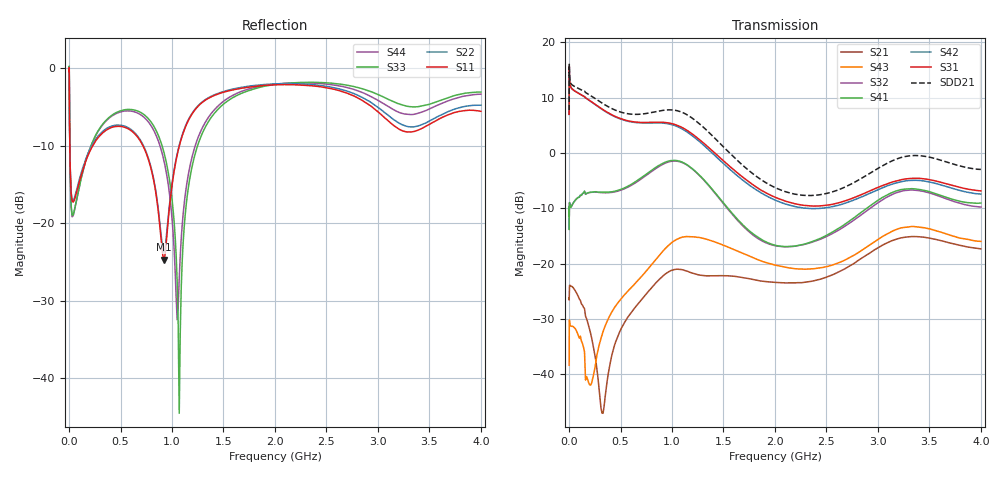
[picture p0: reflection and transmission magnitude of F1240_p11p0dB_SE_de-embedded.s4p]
! Integrated Device Technology
! Corporate Headquarters
! 6024 Silver Creek Valley Road
! San Jose, CA 95138  USA
! Phone:  1-408-284-8200
! Toll Free:  1-800-223-1366
! Webpage:  http://www.idt.com/
! Timing and RF Division
! 515 Groton Road, Suite 102
! Westford, MA 01886-6024
! Device:  F1240
! Description: Dual Intermediate Frequency Digital Variable Gain Amplifier
! Frequency:  10.0 -  500.00 MHz
! Package:  5x5 mm QFN Plastic Package: 32 pin
! Ports:  8 RF, 20 DC
!  Pin  1  = GA3 / Data  Pin 17  = RF OUT_B+
!  Pin  2  = GA4 / CLK  Pin 18  = RF OUT_B-
!  Pin  3  = GA5  Pin 19  = STBY_B
!  Pin  4  = VMODE  Pin 20  = Ground
!  Pin  5  = No Connect  Pin 21  = Ground
!  Pin  6  = GB5  Pin 22  = STB_A
!  Pin  7  = GB4  Pin 23  = RF OUT_A-  = Port 4
!  Pin  8  = GB3  Pin 24  = RF OUT_A+  = Port 3
!  Pin  9  = GB2  Pin 25  = GA0
!  Pin 10  = GB1  Pin 26  = ISET_A
!  Pin 11  = RF IN_B+  Pin 27  = VCC
!  Pin 12  = RF IN_B-  Pin 28  = Ground
!  Pin 13  = Ground  Pin 29  = RF IN_A-  = Port 2
!  Pin 14  = VCC  Pin 30  = RF IN_A+  = Port 1
!  Pin 15  = ISET_B  Pin 31  = GA1
!  Pin 16  = GB0  Pin 32  = GA2 / CSb
! Gain  = +19.5 dB
! State  = 1
! Voltage  = +5.00 V
! Current  = 85.292 mA (one channel only)
! Temperture  =  +25 C
! Test Date  =  2017-10-18
! Board  =  EB4031
! Data:  The device was measured on a custom evaluation board which has
!  individual transmission lines to the RF pins.  Data was collected
!  using a calibrated network analyzer.  The evaluation board was
!  de-embedded using Automatic Fixture Removal.
!  The reference plane is the edge of the package pin.
!  Only Channel A was measured.
!  This data is in single-ended operation.  If your needs are balanced
!  or differential S-parameters then this file needs to be used a
!  linear simulator.
! File Date:  2017-11-10  MJV
! Note:
!  Integrated Device Technology supplies this data as a sample of measured
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# Hz S dB R 100
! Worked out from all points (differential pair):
!   410 points, 500 kHz to 4 GHz, reference 100 ohm
!   strongest paths, dB at 500 kHz, 930 MHz, 1.96 GHz, 2.98 GHz, 4 GHz:
!     S31: 7.0, 5.5, -7.7, -6.4, -6.9
!     S42: 7.0, 5.4, -8.2, -6.8, -7.4
!     S41: -13.8, -1.7, -16.5, -8.8, -9.1
!     S32: -13.7, -1.9, -16.6, -9.3, -9.8
!     S43: -38.4, -17.4, -20.1, -15.9, -16.0
!     S21: -26.2, -22.0, -23.4, -17.4, -17.4
!   taken as a pair (ports 1,2 in; 3,4 out), SDD21 dB: 7.7, 7.8, -5.9, -3.0, -3.0
!   lowest |S11| = -24.7 dB at 920 MHz (marker M1), VSWR 1.12, Z = 110 + j7.17 ohm
!   |S11| at or under -10 dB: 7.642 MHz to 229.3 MHz (221.7 MHz wide, 187 % of centre); 718.6 MHz to 1.071 GHz (352.2 MHz wide, 39.4 % of centre)
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500000  -0.39 -5.8  -26.21 -3.1  -27.23 80.3  -58.76 70.0
        -26.21 -3.2  -0.39 -5.7  -58.61 67.2  -27.24 81.5
        7.01 -105.1  -13.74 67.6  -0.48 1.3  -38.51 -119.2
        -13.82 68.7  6.98 -104.0  -38.41 -118.4  -0.49 3.6
3000000  -3.36 -58.3  -25.29 3.8  -16.83 21.3  -46.59 62.7
         -25.26 3.9  -3.33 -58.3  -46.62 62.9  -16.84 21.5
         14.97 -177.0  -9.80 -4.6  -2.89 -53.9  -30.27 72.8
         -9.72 -4.5  14.96 -176.8  -30.23 72.6  -2.95 -53.7
2e8  -10.75 -128.4  -31.83 -83.9  -19.13 -50.9  -34.22 14.2
     -31.96 -82.2  -10.52 -129.6  -34.21 14.7  -19.15 -51.0
     9.49 109.4  -7.16 -35.4  -10.44 -91.3  -39.84 -152.3
     -7.13 -35.7  9.46 108.7  -41.94 -158.8  -10.46 -90.4
5.3e8  -7.55 -178.7  -31.67 -7.1  -20.48 -107.8  -28.45 -56.6
       -30.96 -10.3  -7.40 -179.9  -28.58 -54.8  -20.62 -108.1
       6.03 26.8  -6.54 -98.9  -5.36 -155.3  -27.03 20.0
       -6.39 -100.4  5.95 25.8  -25.84 15.3  -5.51 -155.2
9.2e8  -24.67 33.8  -22.05 -80.1  -18.22 169.6  -24.69 -148.6
       -22.12 -88.4  -23.69 32.6  -24.98 -142.7  -18.55 169.0
       5.53 -69.7  -1.96 165.8  -10.74 139.0  -18.60 -63.4
       -1.78 161.7  5.40 -71.5  -17.58 -70.0  -11.81 140.8
1.52e9  -2.99 -149.7  -21.68 140.5  -24.27 29.4  -26.36 74.4
        -22.21 143.2  -2.90 -149.5  -26.15 80.2  -25.28 29.2
        -1.77 127.8  -9.65 -16.8  -4.39 -136.7  -17.28 130.2
        -9.49 -22.3  -2.27 126.8  -16.84 127.0  -4.04 -139.7
4e9  -5.53 -153.1  -17.43 72.5  -20.91 -57.5  -20.53 -47.9
     -17.35 72.0  -4.75 -148.9  -22.29 -28.7  -23.41 -49.5
     -6.86 17.1  -9.77 -104.6  -3.05 -138.3  -16.28 88.0
     -9.06 -117.4  -7.44 25.6  -16.00 61.5  -3.31 -144.7
